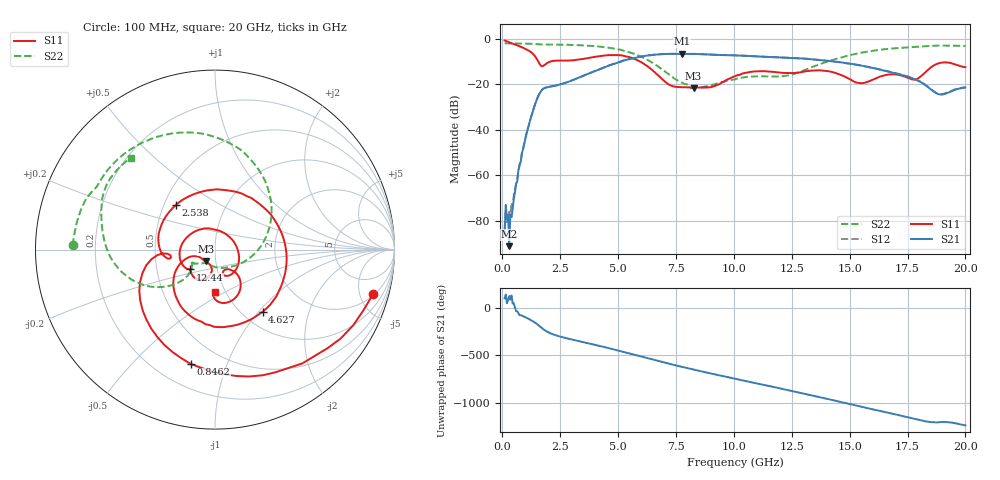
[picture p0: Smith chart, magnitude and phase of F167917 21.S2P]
!  2-Port S-parameters saved by WinCal
! VAR MeasName=S-Parameters (CALIBRATED_DATA) read from VNA (N5242A)
! VAR MeasDate=2016-11-22 9:00:45
! VAR NAME=F167917 21
! VAR FILENAME=F167917 21.S2P
! VAR DATE=2016-11-22 9:00:45
! VAR PHYS_PORTS=1,2
# Hz S DB R 50
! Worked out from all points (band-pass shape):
!   401 points, 100 MHz to 20 GHz, reference 50 ohm
!   highest |S21| = -6.63 dB at 7.761 GHz (marker M1); lowest = -91.2 dB at 299 MHz (marker M2)
!   |S21| within 3 dB of the highest: 5.235 GHz to 13.94 GHz (8.706 GHz wide, 90.8 % of centre)
!   lowest |S11| = -21.7 dB at 8.259 GHz (marker M3), VSWR 1.18, Z = 44.9 - j5.92 ohm
!   |S11| at or under -10 dB: 1.553 GHz to 2.089 GHz (535.6 MHz wide, 29.4 % of centre); 5.944 GHz to end of sweep
!   |S22| runs from -21.4 to -2.0 dB; largest |S21 - S12| = 0.0052
!   S11 on the Smith chart (normalised r, x): 100 MHz: 2.17, -6.62; 846.2 MHz: 0.34, -0.75; 2.538 GHz: 0.58, +0.32; 4.627 GHz: 1.23, -1.05; 12.44 GHz: 0.74, -0.17; 20 GHz: 0.90, -0.45
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1e8  -0.76 -15.6  -86.10 108.3  -83.48 -76.5  -2.03 178.3
2.99e8  -1.58 -41.2  -91.16 131.8  -76.03 84.3  -2.05 175.1
8.4625e8  -3.72 -101.9  -50.29 -75.2  -50.41 -74.9  -2.14 166.4
1.24425e9  -5.93 -145.5  -34.37 -125.3  -34.28 -125.3  -2.23 159.9
1.5925e9  -10.73 -175.8  -24.42 175.4  -24.36 175.4  -2.44 154.2
2.53775e9  -9.61 131.1  -20.01 58.4  -19.96 58.1  -2.59 139.8
3.43325e9  -8.99 45.5  -16.56 5.4  -16.55 5.3  -2.90 121.9
4.62725e9  -7.21 -52.5  -11.71 -63.5  -11.69 -63.5  -4.01 90.9
5.72175e9  -8.94 -124.6  -8.43 -132.9  -8.39 -133.0  -6.75 51.1
6.7665e9  -16.39 -163.9  -6.85 159.8  -6.85 159.6  -12.46 -0.9
7.7615e9  -21.36 -136.6  -6.63 99.0  -6.63 99.1  -19.33 -71.0
8.259e9  -21.73 -127.0  -6.66 70.4  -6.65 70.5  -20.95 -107.3
1.005e10  -16.49 -102.7  -7.33 -27.1  -7.32 -27.0  -17.84 -142.6
1.119425e10  -14.25 -126.0  -7.88 -87.6  -7.86 -87.5  -16.53 -154.2
1.2438e10  -15.08 -141.1  -8.43 -153.2  -8.41 -153.4  -15.85 -143.4
1.338325e10  -14.02 -154.7  -9.04 154.3  -9.03 154.4  -12.43 -136.4
1.4627e10  -15.93 146.5  -10.42 85.3  -10.39 85.1  -8.28 -147.2
1.55225e10  -19.54 54.3  -11.86 34.4  -11.88 34.7  -6.12 -160.3
1.67165e10  -15.71 -49.0  -14.51 -32.3  -14.49 -31.5  -4.41 179.9
1.786075e10  -17.94 -60.4  -18.00 -97.5  -17.89 -96.9  -3.58 163.0
1.885575e10  -10.76 -66.2  -24.44 -129.7  -24.24 -128.9  -3.03 147.8
2e10  -12.52 -89.4  -21.43 -164.1  -21.25 -164.0  -3.16 132.5
